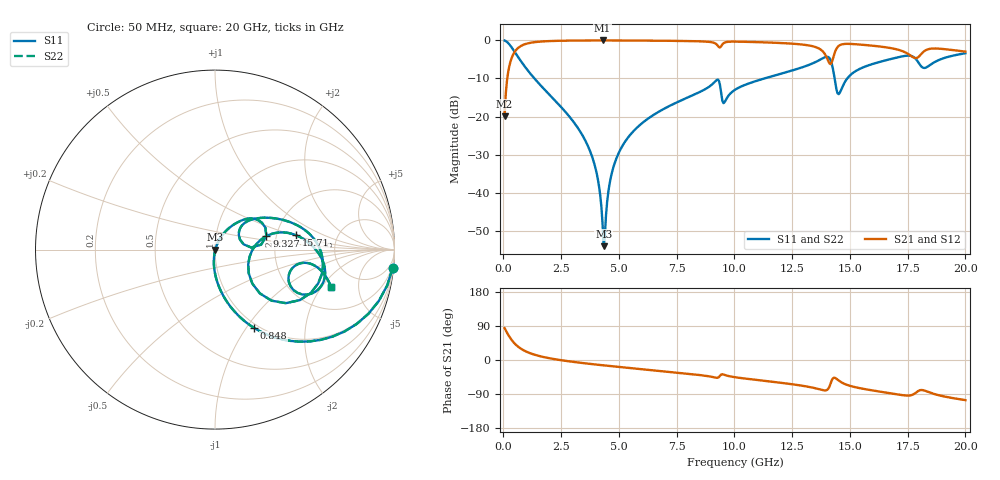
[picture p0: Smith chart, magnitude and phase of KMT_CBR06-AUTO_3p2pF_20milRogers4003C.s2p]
! Data measured by Modelithics Inc. support@modelithics.com 813-866-6335
! KEMET CBR06-AUTO 3.2pF, Pad Width= 0.851mm, Pad Length= 0.64mm, Pad Gap= 0.62mm, 20mil Rogers 4003C substrate Data, January 2022
# hz S ma R 50
! 2 Port Network Data from SP1.SP block
! freq  magS11  angS11  magS21  angS21  magS12  angS12  magS22  angS22
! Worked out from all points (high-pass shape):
!   401 points, 50 MHz to 20 GHz, reference 50 ohm
!   highest |S21| = -0.02 dB at 4.289 GHz (marker M1); lowest = -19.9 dB at 50 MHz (marker M2)
!   |S21| within 3 dB of the highest: 487.3 MHz to 13.84 GHz (13.36 GHz wide, 186 % of centre); 14.36 GHz to 17.35 GHz (2.998 GHz wide, 18.9 % of centre)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
!   lowest |S11| = -54.0 dB at 4.339 GHz (marker M3), VSWR 1.00, Z = 50.2 - j0.121 ohm
!   |S11| at or under -10 dB: 1.342 GHz to 11.29 GHz (9.95 GHz wide, 158 % of centre); 14.34 GHz to 14.88 GHz (547.7 MHz wide, 3.75 % of centre)
!   |S22| runs from -54.0 to 0.0 dB; largest |S21 - S12| = 0
!   S11 on the Smith chart (normalised r, x): 50 MHz: 1, -19; 848 MHz: 0.95, -1.09; 9.327 GHz: 1.77, +0.30; 15.71 GHz: 2.58, +0.52; 20 GHz: 3.22, -2.46
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5e7  0.9949 -6.0  0.1011 84.0  0.1011 84.0  0.9949 -6.0
3.4925e8  0.8135 -36.6  0.5807 53.3  0.5807 53.3  0.8135 -36.6
8.48e8  0.488 -63.5  0.8718 26.4  0.8718 26.4  0.488 -63.5
3.391625e9  0.05885 -96.2  0.9965 -7.7  0.9965 -7.7  0.05885 -96.2
3.990125e9  0.02072 -97.0  0.9979 -11.9  0.9979 -11.9  0.02072 -97.0
4.289375e9  0.003981 -76.6  0.998 -13.8  0.998 -13.8  0.003981 -76.6
4.33925e9  0.001995 -37.3  0.998 -14.2  0.998 -14.2  0.001995 -37.3
4.688375e9  0.01797 67.5  0.9978 -16.4  0.9978 -16.4  0.01797 67.5
5.0375e9  0.03569 68.3  0.9972 -18.5  0.9972 -18.5  0.03569 68.3
6.73325e9  0.1163 60.2  0.9905 -28.6  0.9905 -28.6  0.1163 60.2
9.32675e9  0.2963 15.0  0.8185 -45.1  0.8185 -45.1  0.2963 15.0
9.576125e9  0.1548 30.8  0.9366 -39.4  0.9366 -39.4  0.1548 30.8
1.0025e10  0.225 41.9  0.9636 -45.5  0.9636 -45.5  0.225 41.9
1.336662e10  0.4965 14.3  0.8414 -72.7  0.8414 -72.7  0.4965 14.3
1.396512e10  0.6083 -8.5  0.6237 -80.0  0.6237 -80.0  0.6083 -8.5
1.42145e10  0.4949 -37.1  0.5152 -53.7  0.5152 -53.7  0.4949 -37.1
1.451375e10  0.1967 -11.9  0.845 -54.1  0.845 -54.1  0.1967 -11.9
1.571075e10  0.4598 10.0  0.8674 -77.5  0.8674 -77.5  0.4598 10.0
1.670825e10  0.5634 -0.3  0.7984 -87.5  0.7984 -87.5  0.5634 -0.3
1.755612e10  0.6306 -16.0  0.6536 -93.9  0.6536 -93.9  0.6306 -16.0
1.815462e10  0.4394 -21.4  0.695 -79.5  0.695 -79.5  0.4394 -21.4
2e10  0.6784 -17.7  0.712 -105.9  0.712 -105.9  0.6784 -17.7
